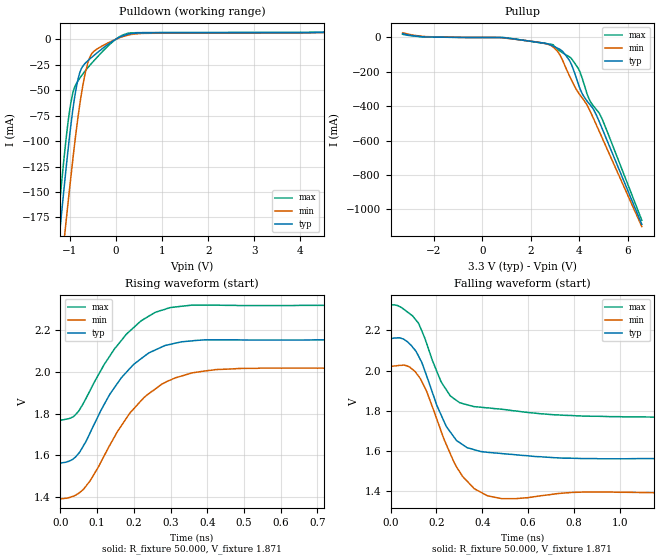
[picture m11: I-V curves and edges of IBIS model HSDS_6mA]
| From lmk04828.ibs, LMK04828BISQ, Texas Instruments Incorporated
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[Model]   HSDS_6mA
Model_type   Output
Polarity   Non-Inverting
Vmeas = 1.9
Vref = 1.9
Cref = 0pF
Rref = 50
|   typ   min   max
|   (nom PVT)   (Fast PVT)   (slow PVT)
C_comp   1.492p   1.392p   1.674p
|C_comp (hi state)   1.492p   1.392p   1.674p
|C_comp (low state)   2.777p   2.419p   2.781p
| Where   nom PVT is  Nominal Process, 3.3V, 27C
|   Fast PVT is Strong Process, 3.45V, -40C
|   Slow PVT is Weak Process, 3.15V, 125C
[Voltage Range]   3.3   3.15   3.45
[Temperature Range]   27   125   -40
[Pullup Reference]   3.3   3.15   3.45
[Pulldown Reference]   0   0   0
[Power Clamp Reference]   3.3   3.15   3.45
[GND Clamp Reference]   0   0   0
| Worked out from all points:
|   slope of the pulldown table from 0 to 0.495 V, typ, clamps not added: 81.8 ohm
|   slope of the pullup table from 0 to 0.495 V, typ, clamps not added: 8 kohm
|   falling waveform, R_fixture 50.000, V_fixture 1.871: 20-80 % time 131ps typ, 131ps min, 127ps max; typ from 2.16 V to 1.56 V
|   rising waveform, R_fixture 50.000, V_fixture 1.871: 20-80 % time 127ps typ, 145ps min, 127ps max; typ from 1.56 V to 2.16 V
[Pulldown]
|   Voltage   I(typ)   I(min)   I(max)
-3.3V     -1.225A    -1.2A      -1.253A
-1.28V    -220mA     -267.9mA   -190.8mA
-1.221V   -191.9mA   -241.5mA   -162.2mA
-1.122V   -146.4mA   -198mA     -116.6mA
-1.073V   -124.5mA   -176.5mA   -95.65mA
-993.3mV  -91.71mA   -143.1mA   -67.69mA
-864.6mV  -49.48mA   -92.41mA   -44.34mA
-755.7mV  -29.9mA    -56.55mA   -36.73mA
-607.2mV  -21.23mA   -23.33mA   -28.05mA
-409.2mV  -13.55mA   -9.712mA   -17.97mA
145.2mV   3.146mA    2.35mA     3.956mA
6.59V     8.158mA    8.228mA    8.143mA
[Pullup]
|   Voltage   I(typ)   I(min)   I(max)
-3.3V     22.29mA    27.13mA    18.75mA
-2.35V    3.194mA    4.974mA    2.65mA
887.7mV   -1.305mA   -2.825mA   -285.8uA
2.363V    -29.22mA   -28.44mA   -30.16mA
2.907V    -48.93mA   -53.53mA   -41.57mA
3.303V    -79.32mA   -129.3mA   -88.07mA
3.679V    -156.4mA   -246.4mA   -122.6mA
3.986V    -278.6mA   -324.7mA   -186.1mA
4.412V    -384.7mA   -416.3mA   -358.4mA
4.709V    -450.1mA   -507.4mA   -418.8mA
4.957V    -531.6mA   -585.6mA   -475.6mA
6.59V     -1.086A    -1.1A      -1.063A
[Ramp]
R_load = 50
|   typ   min   max
dV/dt_r   0.350058/1.26814e-10   0.377034/1.45031e-10   0.33351/1.26836e-10
dV/dt_f   0.350156/1.31831e-10   0.377034/1.30965e-10   0.333973/1.27082e-10
[Falling Waveform]
R_fixture = 50.000
V_fixture = 1.871
V_fixture_min = 1.682
V_fixture_max = 2.094
C_fixture = 0.000
|  time   V(typ)   V(min)   V(max)
|   0.000S   2.157V   2.019V   2.324V
|  161.057ps   2.157V   2.019V   2.324V
|  164.914ps   2.157V   2.019V   2.324V
|  170.432ps   2.157V   2.019V   2.324V
|  195.552ps   2.157V   2.020V   2.324V
|  216.389ps   2.158V   2.020V   2.325V
|  222.292ps   2.158V   2.020V   2.325V
|  223.394ps   2.159V   2.020V   2.325V
|  234.419ps   2.159V   2.020V   2.326V
|  243.455ps   2.160V   2.021V   2.327V
|  245.267ps   2.160V   2.021V   2.327V
|  246.322ps   2.160V   2.021V   2.327V
|  253.000ps   2.161V   2.022V   2.327V
|  259.299ps   2.162V   2.023V   2.327V
|  261.074ps   2.162V   2.023V   2.326V
|  264.622ps   2.162V   2.023V   2.326V
|  266.701ps   2.162V   2.024V   2.325V
|  271.718ps   2.163V   2.024V   2.324V
|  277.114ps   2.163V   2.025V   2.321V
|  280.348ps   2.163V   2.026V   2.319V
|  284.057ps   2.162V   2.026V   2.317V
|  284.179ps   2.162V   2.026V   2.317V
|  291.533ps   2.159V   2.026V   2.312V
|  294.967ps   2.158V   2.027V   2.309V
|  295.198ps   2.158V   2.027V   2.309V
|  297.001ps   2.157V   2.027V   2.307V
|  299.256ps   2.156V   2.027V   2.305V
|  302.529ps   2.153V   2.026V   2.303V
|  307.836ps   2.149V   2.025V   2.298V
|  313.340ps   2.145V   2.023V   2.293V
|  317.114ps   2.141V   2.021V   2.290V
|  324.995ps   2.132V   2.017V   2.283V
|  331.859ps   2.125V   2.010V   2.277V
|  337.826ps   2.116V   2.005V   2.272V
|  348.177ps   2.102V   1.995V   2.257V
|  353.316ps   2.094V   1.987V   2.250V
|  363.833ps   2.071V   1.971V   2.235V
|  372.233ps   2.052V   1.958V   2.212V
|  378.153ps   2.039V   1.944V   2.196V
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0s        2.157V     2.019V     2.324V
71.72ps   2.145V     2.023V     2.293V
130.6ps   2.052V     1.958V     2.212V
220.1ps   1.779V     1.698V     1.944V
260ps     1.694V     1.586V     1.874V
314.7ps   1.63V      1.471V     1.835V
364.5ps   1.605V     1.411V     1.82V
484.5ps   1.586V     1.361V     1.807V
958.4ps   1.56V      1.394V     1.77V
2.758ns   1.562V     1.391V     1.767V
[Rising Waveform]
R_fixture = 50.000
V_fixture = 1.871
V_fixture_min = 1.682
V_fixture_max = 2.094
C_fixture = 0.000
|  time   V(typ)   V(min)   V(max)
|   0.000S   1.562V   1.391V   1.767V
|  159.494ps   1.562V   1.391V   1.767V
|  160.227ps   1.562V   1.391V   1.767V
|  161.057ps   1.562V   1.391V   1.767V
|  195.552ps   1.562V   1.391V   1.767V
|  202.771ps   1.562V   1.391V   1.767V
|  221.693ps   1.562V   1.391V   1.768V
|  229.502ps   1.562V   1.391V   1.768V
|  231.184ps   1.562V   1.391V   1.768V
|  234.419ps   1.562V   1.391V   1.768V
|  234.547ps   1.562V   1.391V   1.768V
|  239.644ps   1.562V   1.391V   1.769V
|  240.380ps   1.562V   1.391V   1.769V
|  243.455ps   1.563V   1.391V   1.769V
|  246.322ps   1.563V   1.391V   1.770V
|  253.000ps   1.565V   1.392V   1.771V
|  257.576ps   1.566V   1.393V   1.773V
|  257.638ps   1.566V   1.393V   1.773V
|  259.299ps   1.567V   1.393V   1.773V
|  264.413ps   1.570V   1.395V   1.775V
|  264.622ps   1.570V   1.395V   1.775V
|  266.701ps   1.571V   1.396V   1.776V
|  271.518ps   1.575V   1.398V   1.779V
|  271.718ps   1.575V   1.398V   1.779V
|  273.643ps   1.577V   1.400V   1.781V
|  277.114ps   1.580V   1.402V   1.784V
|  280.348ps   1.585V   1.404V   1.787V
|  284.057ps   1.590V   1.407V   1.794V
|  284.179ps   1.590V   1.407V   1.794V
|  291.533ps   1.605V   1.415V   1.808V
|  294.967ps   1.612V   1.419V   1.816V
|  295.198ps   1.613V   1.419V   1.817V
|  297.001ps   1.617V   1.422V   1.822V
|  299.256ps   1.624V   1.425V   1.829V
|  302.529ps   1.633V   1.430V   1.838V
|  307.836ps   1.650V   1.439V   1.855V
|  313.340ps   1.666V   1.451V   1.873V
|  317.114ps   1.680V   1.460V   1.886V
|  324.995ps   1.709V   1.478V   1.913V
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0s        1.562V     1.391V     1.767V
36.5ps    1.585V     1.404V     1.787V
63.99ps   1.65V      1.439V     1.855V
88.01ps   1.735V     1.498V     1.937V
134.3ps   1.893V     1.648V     2.077V
199.4ps   2.037V     1.823V     2.214V
257.8ps   2.106V     1.918V     2.287V
287.5ps   2.129V     1.953V     2.304V
422.2ps   2.155V     2.012V     2.322V
2.756ns   2.157V     2.019V     2.323V
